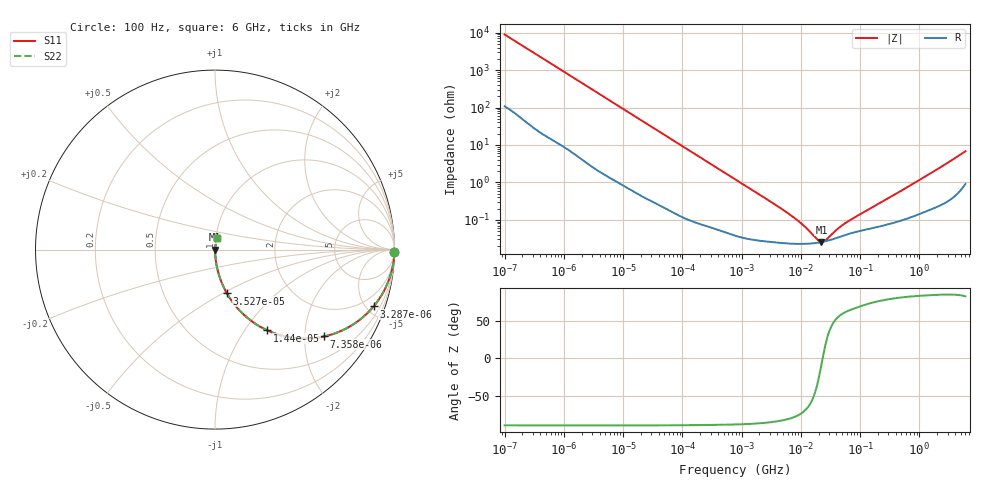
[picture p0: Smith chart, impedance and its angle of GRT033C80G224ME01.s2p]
!Murata Part Number: GRT033C80G224ME01
!These Parameters are Measured in Series Mode Connection
!Data Generated on Jun 19, 2026
!  o--ll--o
!Port1  Port2
!  o------o
!Operation Temp=25[degC], DC Bias Voltage=0[V]
!Freq. Start=100[Hz] Stop=6[GHz] 401[Steps]
# Hz S RI R 50
!Freq.(Hz) S11(Real) S11(Imag) S21(Real) S21(Imag) S12(Real) S12(Imag) S22(Real) S22(Imag)
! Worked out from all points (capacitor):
!   401 points, 100 Hz to 6 GHz, reference 50 ohm
!   read as one part in series: C = 177 nF near 109 Hz
!   lowest |Z| = 25.8 mohm at 22.26 MHz (marker M1)
!   series resonance near 23.37 MHz, so ESL is about 260 pH
!   S11 on the Smith chart (normalised r, x): 100 Hz: open; 3.287 kHz: 1.05, -5.56; 7.358 kHz: 1.02, -2.49; 14.4 kHz: 1.01, -1.28; 35.27 kHz: 1.01, -0.53; 6 GHz: 1.02, +0.13
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100  0.9997 -0.0112  0.00026 0.0112  0.00026 0.0112  0.9997 -0.0112
600  0.995 -0.0659  0.00499 0.0659  0.00499 0.0659  0.995 -0.0659
2008  0.9521 -0.2092  0.0479 0.2092  0.0479 0.2092  0.9521 -0.2092
3287  0.8835 -0.3166  0.1165 0.3166  0.1165 0.3166  0.8835 -0.3166
4918  0.7744 -0.4138  0.2256 0.4138  0.2256 0.4138  0.7744 -0.4138
7358  0.6079 -0.4839  0.3921 0.4839  0.3921 0.4839  0.6079 -0.4839
14402  0.2921 -0.4502  0.7079 0.4502  0.7079 0.4502  0.2921 -0.4502
22537  0.1462 -0.3485  0.8538 0.3485  0.8538 0.3485  0.1462 -0.3485
35265  0.0667 -0.2443  0.9333 0.2443  0.9333 0.2443  0.0667 -0.2443
40335  0.0523 -0.2172  0.9477 0.2172  0.9477 0.2172  0.0523 -0.2172
129199  0.00616 -0.0717  0.9938 0.0717  0.9938 0.0717  0.00616 -0.0717
774597  0.000526 -0.0122  0.9995 0.0122  0.9995 0.0122  0.000526 -0.0122
6353432  0.000234 -0.00141  0.9998 0.00141  0.9998 0.00141  0.000234 -0.00141
1.039699e7  0.000228 -0.000745  0.9998 0.000745  0.9998 0.000745  0.000228 -0.000745
1.555665e7  0.000235 -0.000343  0.9998 0.000343  0.9998 0.000343  0.000235 -0.000343
1.946e7  0.000245 -0.00015  0.9998 0.00015  0.9998 0.00015  0.000245 -0.00015
2.225763e7  0.000255 -3.93e-05  0.9997 3.93e-05  0.9997 3.93e-05  0.000255 -3.93e-05
2.662322e7  0.000271 0.000104  0.9997 -0.000104  0.9997 -0.000104  0.000271 0.000104
4.165952e7  0.000334 0.000461  0.9997 -0.000461  0.9997 -0.000461  0.000334 0.000461
5.960426e7  0.000405 0.000765  0.9996 -0.000765  0.9996 -0.000765  0.000405 0.000765
3.124326e8  0.00079 0.00383  0.9992 -0.00383  0.9992 -0.00383  0.00079 0.00383
6e9  0.0134 0.0658  0.9866 -0.0658  0.9866 -0.0658  0.0134 0.0658
